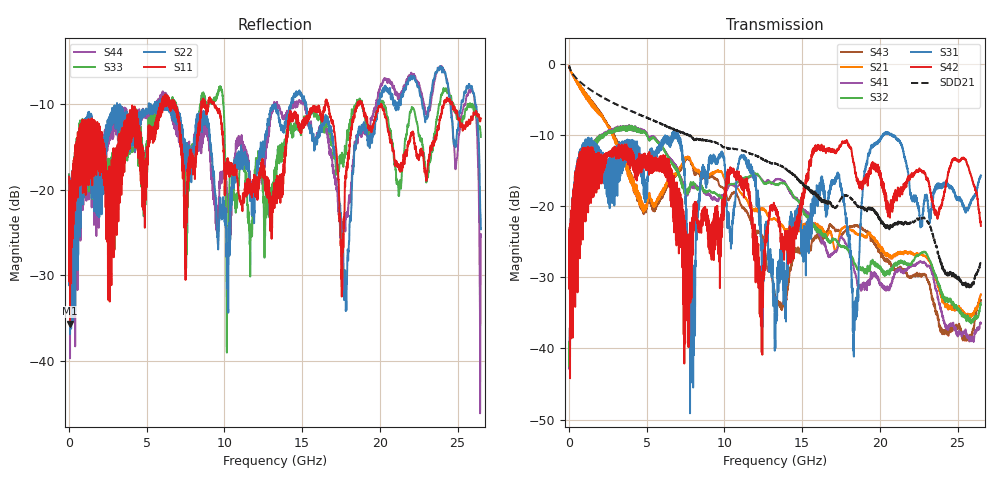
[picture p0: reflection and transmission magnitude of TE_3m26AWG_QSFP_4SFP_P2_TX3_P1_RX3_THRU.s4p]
!Agilent Technologies,N5222A,MY51421691,A.10.00.00
!Agilent N5222A: A.10.00.00
!Date: Friday, January 30, 2015 12:33:38
!Correction: S11(Full 4 Port(1,2,3,4))
!S12(Full 4 Port(1,2,3,4))
!S13(Full 4 Port(1,2,3,4))
!S14(Full 4 Port(1,2,3,4))
!S21(Full 4 Port(1,2,3,4))
!S22(Full 4 Port(1,2,3,4))
!S23(Full 4 Port(1,2,3,4))
!S24(Full 4 Port(1,2,3,4))
!S31(Full 4 Port(1,2,3,4))
!S32(Full 4 Port(1,2,3,4))
!S33(Full 4 Port(1,2,3,4))
!S34(Full 4 Port(1,2,3,4))
!S41(Full 4 Port(1,2,3,4))
!S42(Full 4 Port(1,2,3,4))
!S43(Full 4 Port(1,2,3,4))
!S44(Full 4 Port(1,2,3,4))
!S4P File: Measurements: <S11,S12,S13,S14>,
!<S21,S22,S23,S24>,
!<S31,S32,S33,S34>,
!<S41,S42,S43,S44>:
# Hz S  dB  R 50.0
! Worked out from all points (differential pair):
!   2650 points, 10 MHz to 26.5 GHz, reference 50 ohm
!   strongest paths, dB at 10 MHz, 6.63 GHz, 13.26 GHz, 19.88 GHz, 26.5 GHz:
!     S42: -24.9, -15.9, -20.1, -14.2, -22.8
!     S31: -25.0, -10.3, -34.7, -10.8, -15.7
!     S32: -39.5, -14.0, -16.9, -28.4, -33.6
!     S41: -39.6, -13.7, -16.3, -30.0, -36.4
!     S21: -0.4, -15.7, -21.8, -25.5, -32.4
!     S43: -0.4, -16.1, -32.6, -26.3, -33.2
!   taken as a pair (ports 1,3 in; 2,4 out), SDD21 dB: -0.3, -9.1, -14.0, -21.5, -27.9
!   lowest |S11| = -35.7 dB at 70 MHz (marker M1), VSWR 1.03, Z = 51.4 + j0.849 ohm
!   |S11| at or under -10 dB: start of sweep to 5.869 GHz; 9.338 GHz to 16.5 GHz (7.159 GHz wide, 55.4 % of centre); 20.09 GHz to 24.12 GHz (4.03 GHz wide, 18.2 % of centre)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
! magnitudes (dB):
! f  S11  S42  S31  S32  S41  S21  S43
! 10 MHz  -18.5  -24.9  -25.0  -39.5  -39.6  -0.4  -0.4
! 70 MHz  -35.7  -44.2  -39.7  -38.4  -38.6  -0.8  -0.8
! 3.92 GHz  -10.7  -12.0  -10.8  -9.2  -9.2  -15.8  -15.5
! 12.36 GHz  -17.7  -33.1  -23.6  -16.2  -16.1  -20.3  -23.8
! 18.39 GHz  -10.7  -14.8  -33.4  -28.2  -29.4  -23.8  -22.8
! 19.53 GHz  -12.7  -14.2  -11.8  -27.5  -29.4  -24.3  -24.8
! 26.5 GHz  -11.7  -22.8  -15.7  -33.6  -36.4  -32.4  -33.2
